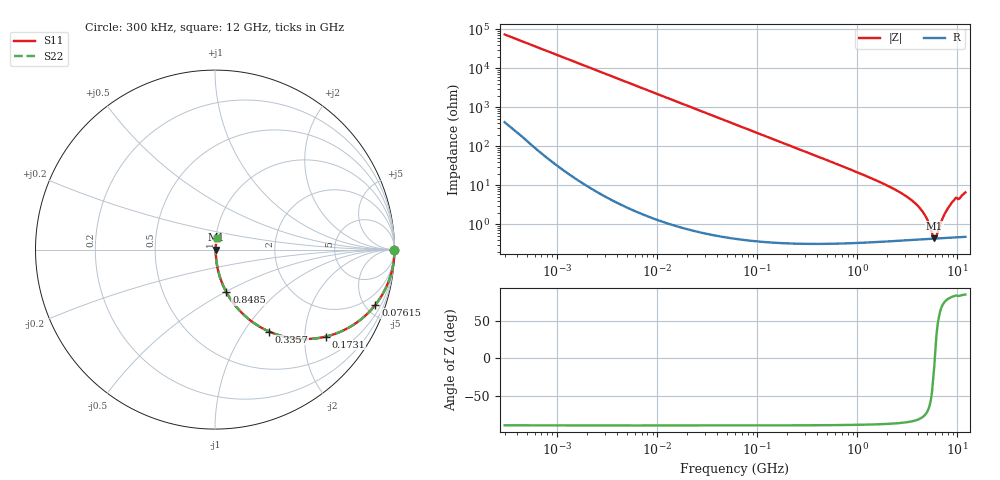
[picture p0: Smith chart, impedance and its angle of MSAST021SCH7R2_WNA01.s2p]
! MSAST021SCH7R2_WNA01  S-PARAMETER MODEL  ( General Type )
! Model Generated by TAIYO YUDEN Corporation (http://www.ty-top.com)
! Version 2.0
! TAIYO YUDEN Control No. 181101
! Copyright(c) 2015 TAIYO YUDEN CO.,LTD. All Rights Reserved.
! Product Description (link to TY-COMPAS)
! https://ds.yuden.co.jp/TYCOMPAS/or/detail?pn=MSAST021SCH7R2CWNA01&u=M
! Products Name : Multilayer Ceramic Capacitors
! Characteristics :
!  Capacitance : 7.2 pF , Rated Voltage : 25V , TCC : CH / C0H
!  Case Size : 0.25 x 0.125 / 0.0098 x 0.0049 [mm/inch] , Thickness : 0.125 / 0.0049 [mm/inch]
!  (Conditions: Temperature = 25 degC , DC Bias Current/Voltage = 0A / 0V)
! External Node Assignments :
!  1  o---| |---o  2
! GND o---------o GND
! Frequency Range : 0.3MHz  -  12000MHz  [ 401 STEP ]
# MHz S RI R 50
! Freq[MHz].  S11 Real  S11 Imag  S21 Real  S21 Imag  S12 Real  S12 Imag  S22 Real  S22 Imag
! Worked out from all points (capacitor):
!   401 points, 300 kHz to 12 GHz, reference 50 ohm
!   read as one part in series: C = 7.2 pF near 316.3 kHz
!   lowest |Z| = 437 mohm at 5.869 GHz (marker M1)
!   series resonance near 5.94 GHz, so ESL is about 100 pH
!   S11 on the Smith chart (normalised r, x): 300 kHz: open; 76.15 MHz: 1.01, -5.80; 173.1 MHz: 1.01, -2.55; 335.7 MHz: 1.01, -1.31; 848.5 MHz: 1.01, -0.51; 12 GHz: 1.01, +0.13
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0.3  1 -0.00136  9.49e-06 0.00136  9.49e-06 0.00136  1 -0.00136
1.769972  0.9999 -0.00801  7.15e-05 0.00801  7.15e-05 0.00801  0.9999 -0.00801
10.44266  0.9977 -0.0471  0.00225 0.0471  0.00225 0.0471  0.9977 -0.0471
27.10171  0.9851 -0.1208  0.0149 0.1208  0.0149 0.1208  0.9851 -0.1208
60  0.9311 -0.2527  0.0689 0.2527  0.0689 0.2527  0.9311 -0.2527
76.15486  0.8935 -0.3077  0.1065 0.3077  0.1065 0.3077  0.8935 -0.3077
173.124  0.6191 -0.4843  0.3809 0.4843  0.3809 0.4843  0.6191 -0.4843
335.7268  0.3019 -0.4567  0.6981 0.4567  0.6981 0.4567  0.3019 -0.4567
353.9943  0.2801 -0.4465  0.7199 0.4465  0.7199 0.4465  0.2801 -0.4465
540.8523  0.143 -0.3462  0.857 0.3462  0.857 0.3462  0.143 -0.3462
848.5281  0.0638 -0.2381  0.9362 0.2381  0.9362 0.2381  0.0638 -0.2381
2088.533  0.012 -0.0911  0.988 0.0911  0.988 0.0911  0.012 -0.0911
3107.553  0.00647 -0.0508  0.9935 0.0508  0.9935 0.0508  0.00647 -0.0508
4050.141  0.00486 -0.0285  0.9951 0.0285  0.9951 0.0285  0.00486 -0.0285
4875.354  0.00436 -0.0142  0.9956 0.0142  0.9956 0.0142  0.00436 -0.0142
5565.855  0.00426 -0.00426  0.9957 0.00426  0.9957 0.00426  0.00426 -0.00426
5868.704  0.00428 -0.000789  0.9957 0.000789  0.9957 0.000789  0.00428 -0.000789
6188.031  0.00432 0.00285  0.9957 -0.00285  0.9957 -0.00285  0.00432 0.00285
7254.098  0.00465 0.0153  0.9953 -0.0153  0.9953 -0.0153  0.00465 0.0153
8503.825  0.0055 0.0311  0.9945 -0.0311  0.9945 -0.0311  0.0055 0.0311
9454.42  0.00659 0.0445  0.9934 -0.0445  0.9934 -0.0445  0.00659 0.0445
12000  0.00895 0.0646  0.991 -0.0646  0.991 -0.0646  0.00895 0.0646
